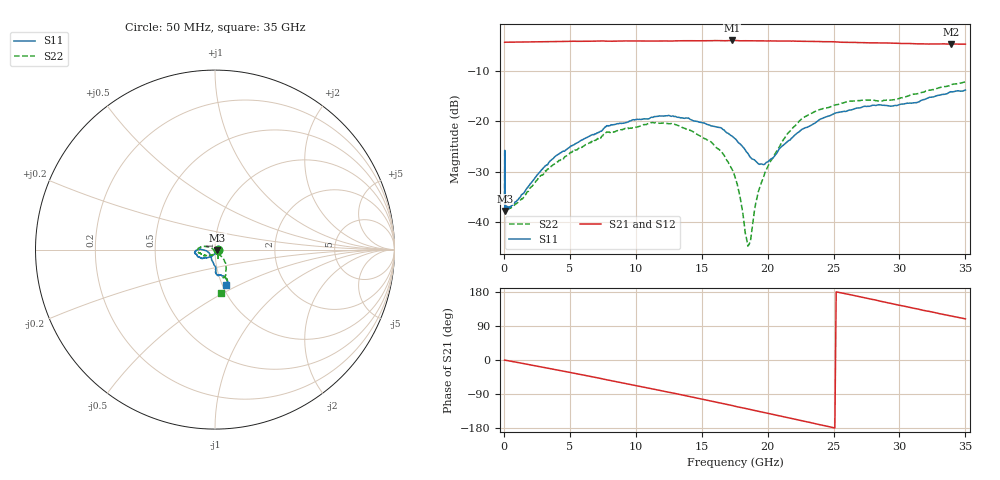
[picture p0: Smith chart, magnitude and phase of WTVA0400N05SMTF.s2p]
! 50 ohm 2-Port S-parameters measured by Modelithics Inc support@modelithics.com  Tampa, FL USA 813-866-6335 (February 2024)
! Smiths Interconnect,  4dB P/N: WTVA0400N05SMTF, Temperature: 25C
! Board: 10 mil Rogers 4350B, Mounting Pad Dimensions: Length: 15 mils, Width: 25 mils, Gap: 40 mils.
# Hz S MA R 50
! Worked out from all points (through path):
!   486 points, 50 MHz to 35 GHz, reference 50 ohm
!   highest |S21| = -3.95 dB at 17.3 GHz (marker M1); lowest = -4.7 dB at 33.9 GHz (marker M2)
!   group delay of S21, straight-line fit = 20.1 ps
!   lowest |S11| = -37.7 dB at 90 MHz (marker M3), VSWR 1.03, Z = 51.3 - j0.208 ohm
!   |S11| at or under -10 dB: start of sweep to end of sweep
!   |S22| runs from -44.7 to -12.2 dB; largest |S21 - S12| = 0.014
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5e7  0.01638 -10.5  0.6094 -0.3  0.6094 -0.3  0.01493 -3.5
8e7  0.016 -14.7  0.61 -0.4  0.609 -0.5  0.01575 -4.6
9e7  0.01298 -9.0  0.6099 -0.5  0.6095 -0.5  0.01332 -8.1
6.5e8  0.01486 -46.9  0.6109 -4.0  0.6107 -4.0  0.01435 -45.4
3.55e9  0.04116 -116.9  0.6178 -22.9  0.6176 -22.9  0.0355 -121.2
5.9e9  0.06579 -135.7  0.6225 -38.9  0.6225 -38.8  0.05531 -143.1
7.8e9  0.09083 -147.3  0.6241 -52.2  0.6239 -52.2  0.07865 -157.2
1.17e10  0.1126 -168.8  0.6271 -79.3  0.627 -79.2  0.0969 -177.2
1.31e10  0.1105 -174.6  0.629 -89.2  0.6287 -89.2  0.0925 175.1
1.56e10  0.09207 179.1  0.6312 -107.4  0.6309 -107.5  0.06399 164.6
1.73e10  0.07173 -179.7  0.6346 -120.1  0.6342 -120.0  0.03371 157.0
1.76e10  0.06637 -178.6  0.6337 -122.8  0.6336 -122.5  0.02618 156.6
1.84e10  0.04986 -173.5  0.6303 -128.5  0.6302 -128.4  0.006902 -161.2
1.86e10  0.04591 -170.2  0.6299 -130.0  0.6295 -129.9  0.006078 -116.5
1.93e10  0.0381 -154.5  0.6286 -135.3  0.6282 -135.2  0.02023 -58.2
2e10  0.03972 -133.0  0.627 -140.5  0.6271 -140.2  0.03566 -50.0
2.16e10  0.0648 -103.8  0.6261 -152.6  0.6259 -152.4  0.07798 -49.1
2.34e10  0.09337 -89.1  0.6221 -166.3  0.6223 -166.1  0.1217 -59.3
2.53e10  0.1226 -88.1  0.6132 179.1  0.6125 179.2  0.1471 -66.0
2.92e10  0.1425 -80.7  0.5981 150.4  0.5979 151.0  0.1621 -71.3
3.39e10  0.197 -68.5  0.5811 116.5  0.5853 116.6  0.2289 -75.9
3.5e10  0.2049 -72.9  0.5837 108.6  0.5831 108.9  0.2455 -82.1
